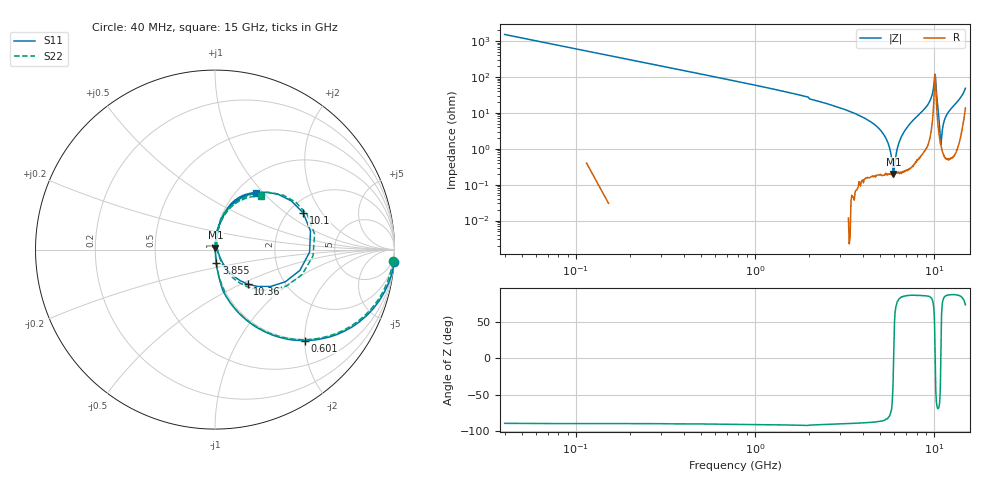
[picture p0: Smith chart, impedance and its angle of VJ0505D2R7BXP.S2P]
! VJ0505D2R7BXP
! MLCC placed on 25 mil thick microstrip substrate in series configuraton.
! DATE 06/29/2018  07:41
! CORRECTED  DATA
# GHz  S  MA  R  50.00
!  FREQ  S11M  S11A  S21M  S21A  S12M  S12A  S22M  S22A
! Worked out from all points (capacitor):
!   401 points, 40 MHz to 15 GHz, reference 50 ohm
!   read as one part in series: C = 2.64 pF near 114.8 MHz
!   lowest |Z| = 198 mohm at 5.949 GHz (marker M1)
!   series resonance near 5.956 GHz, so ESL is about 270 pH
!   S11 on the Smith chart (normalised r, x): 40 MHz: -1, -30; 601 MHz: 0.97, -2.00; 3.855 GHz: 1.00, -0.15; 10.1 GHz: 2.38, +1.36; 10.36 GHz: 1.32, -0.55; 15 GHz: 1.22, +0.92
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0.04  1.001 -3.8  0.0657 85.9  0.06639 86.0  0.9937 -3.7
0.2644  0.9204 -23.7  0.4021 66.4  0.4024 66.5  0.9128 -23.6
0.601  0.7125 -45.4  0.7127 45.4  0.7135 45.4  0.7072 -45.2
1.2742  0.4175 -66.8  0.9205 24.9  0.9211 24.9  0.416 -66.7
2.5458  0.1698 -81.3  0.988 10.4  0.9887 10.5  0.1703 -80.5
3.8548  0.07425 -84.0  0.9956 5.2  0.9961 5.2  0.07455 -84.5
5.0516  0.0225 -82.9  0.9971 2.4  0.9977 2.4  0.02224 -85.0
5.3882  0.009567 -76.7  0.9972 1.7  0.9978 1.7  0.009501 -78.9
5.65  0.002035 -0.5  0.9974 1.2  0.998 1.2  0.001024 8.6
5.9492  0.01102 80.8  0.9974 0.6  0.9977 0.7  0.01094 84.5
6.4728  0.02854 85.6  0.9967 -0.4  0.9973 -0.4  0.02848 86.8
7.52  0.06631 85.9  0.9938 -2.6  0.9945 -2.6  0.06733 84.7
9.5396  0.2188 74.2  0.954 -11.7  0.9547 -11.7  0.2252 72.1
9.8388  0.3243 62.9  0.8864 -17.8  0.8869 -17.8  0.3344 60.6
10.0258  0.4693 40.8  0.6941 -24.3  0.6952 -24.3  0.4863 38.5
10.1006  0.5321 22.7  0.5288 -19.9  0.5289 -19.9  0.55 20.4
10.2502  0.4312 -24.6  0.64 19.1  0.6407 19.1  0.4472 -26.9
10.3624  0.265 -46.6  0.8464 14.9  0.8471 14.9  0.2751 -49.0
10.886  0.01385 5.1  0.9851 0.9  0.9858 1.0  0.01328 -2.1
11.4096  0.06456 83.6  0.9913 -2.9  0.9915 -2.9  0.06592 80.0
12.5316  0.1348 81.0  0.9847 -7.2  0.9852 -7.2  0.1397 80.2
15  0.3921 53.9  0.8151 -22.2  0.8153 -22.2  0.3946 49.1
